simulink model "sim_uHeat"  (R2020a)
settings: Solver=ode15s  StartTime=0.0  StopTime=tsim  MaxStep=1  RelTol=1e-3
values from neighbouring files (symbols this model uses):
  dnom = [T0nom; TDnom; qDnom; Qnom]    [runTransformedMVs.m]
  Kc = 1./(tauC+theta)    [runTransformedMVs.m]
  p1 = [V1;V2;rho;cp;A1;A2;tau01; tau02;transf1]    [runTransformedMVs.m]
  p2 = [V1;V2;rho;cp;A1;A2;tau01; tau02;transf2]    [runTransformedMVs.m]
  T2nom = 30    [runTransformedMVs.m]
  tauI = 4.*(tauC+theta)    [runTransformedMVs.m]
  Tnom = [T1nom;T2nom]    [runTransformedMVs.m]
  umax = 3*Qnom    (= 5016)    [runTransformedMVs.m]
  vbias = [0;0]    [runTransformedMVs.m]
undefined symbols (not defined in the file or in its folder): CalcBlock1, CalcBlock2, Tank

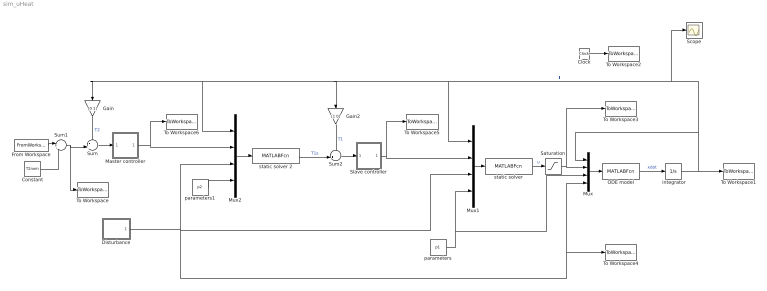
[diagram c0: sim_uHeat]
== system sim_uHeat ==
  " integrator" : Integrator  InitialCondition=Tnom
  Clock : Clock
  Constant : Constant  Value=T2nom
  Disturbance : Subsystem
  From Workspace : FromWorkspace  VariableName=T2sp  OutputAfterFinalValue=Setting to zero
  Gain : Gain  Gain=[0 1]  Multiplication=Matrix(K*u)
  Gain2 : Gain  Gain=[1 0]  Multiplication=Matrix(K*u)
  Master controller : Subsystem
  Mux : Mux
  Mux1 : Mux
  Mux2 : Mux
  ODE model : MATLABFcn  MATLABFcn=Tank(u(1:2), u(3),u(4:12),u(13:16))  OutputDimensions=2
  Saturation : Saturate  UpperLimit=umax  LowerLimit=0
  Scope : Scope
  Slave controller : Subsystem
  Sum : Sum  Inputs=-+|
  Sum1 : Sum  Inputs=|++
  Sum2 : Sum  Inputs=-+|
  To Workspace : ToWorkspace  VariableName=Tsp  SampleTime=-1
  To Workspace1 : ToWorkspace  VariableName=T  SampleTime=-1
  To Workspace2 : ToWorkspace  VariableName=time  SampleTime=-1
  To Workspace3 : ToWorkspace  VariableName=u  SampleTime=-1
  To Workspace4 : ToWorkspace  VariableName=d  SampleTime=-1
  To Workspace5 : ToWorkspace  VariableName=v1  SampleTime=-1
  To Workspace6 : ToWorkspace  VariableName=v2  SampleTime=-1
  parameters : Constant  Value=p1
  parameters1 : Constant  Value=p2
  static solver : MATLABFcn  MATLABFcn=CalcBlock1(u(1:2),u(3),u(4:7),u(8:16))  OutputDimensions=1
  static solver 2 : MATLABFcn  MATLABFcn=CalcBlock2(u(1:2),u(3),u(4:7),u(8:16))  OutputDimensions=1
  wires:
  " integrator"/1 -> Mux/1, Scope/1, Gain/1, Mux2/1, Gain2/1, Mux1/1, To Workspace1/1  "T"
  Mux/1 -> ODE model/1
  Clock/1 -> To Workspace2/1
  static solver/1 -> Saturation/1  "u"
  Mux1/1 -> static solver/1
  ODE model/1 -> " integrator"/1  "xdot"
  parameters/1 -> Mux/3, Mux1/4
  Saturation/1 -> Mux/2, To Workspace3/1
  Disturbance/1(d) -> To Workspace4/1, Mux/4, Mux1/3, Mux2/3
  Mux2/1 -> static solver 2/1
  static solver 2/1 -> Sum2/2  "T1s"
  Sum/1 -> Master controller/1(In1)
  Master controller/1(Out1) -> Mux2/2, To Workspace6/1
  Sum2/1 -> Slave controller/1(In1)
  Slave controller/1(Out1) -> Mux1/2, To Workspace5/1
  Sum1/1 -> Sum/2, To Workspace/1
  Gain/1 -> Sum/1  "T2"
  Gain2/1 -> Sum2/1  "T1"
  parameters1/1 -> Mux2/4
  From Workspace/1 -> Sum1/1
  Constant/1 -> Sum1/2

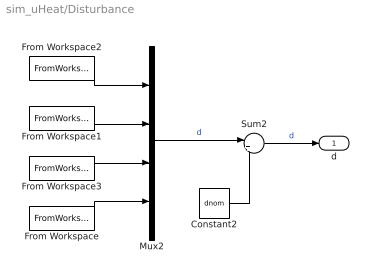
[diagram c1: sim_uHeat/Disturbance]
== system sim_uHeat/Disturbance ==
  Constant2 : Constant  Value=dnom
  From Workspace : FromWorkspace  VariableName=dist{4}  OutputAfterFinalValue=Setting to zero
  From Workspace1 : FromWorkspace  VariableName=dist{2}  OutputAfterFinalValue=Setting to zero
  From Workspace2 : FromWorkspace  VariableName=dist{1}  OutputAfterFinalValue=Setting to zero
  From Workspace3 : FromWorkspace  VariableName=dist{3}  OutputAfterFinalValue=Setting to zero
  Mux2 : Mux
  Sum2 : Sum  Inputs=|++
  d : Outport
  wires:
  From Workspace2/1 -> Mux2/1
  From Workspace/1 -> Mux2/4
  From Workspace3/1 -> Mux2/3
  Mux2/1 -> Sum2/1  "d"
  Constant2/1 -> Sum2/2
  From Workspace1/1 -> Mux2/2
  Sum2/1 -> d/1  "d"

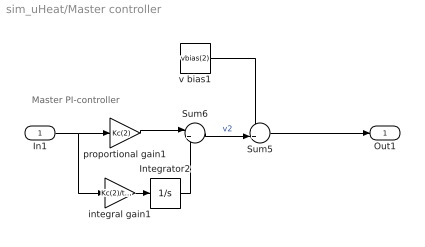
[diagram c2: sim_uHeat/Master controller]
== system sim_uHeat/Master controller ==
  note: Master PI-controller
  In1 : Inport
  Integrator2 : Integrator
  Sum5 : Sum  Inputs=++|
  Sum6 : Sum  Inputs=|++
  integral gain1 : Gain  Gain=Kc(2)/tauI(2)  Multiplication=Matrix(K*u)
  proportional gain1 : Gain  Gain=Kc(2)  Multiplication=Matrix(K*u)
  v bias1 : Constant  Value=vbias(2)
  Out1 : Outport
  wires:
  proportional gain1/1 -> Sum6/1
  Sum6/1 -> Sum5/2  "v2"
  Integrator2/1 -> Sum6/2
  In1/1 -> integral gain1/1, proportional gain1/1
  integral gain1/1 -> Integrator2/1
  Sum5/1 -> Out1/1
  v bias1/1 -> Sum5/1

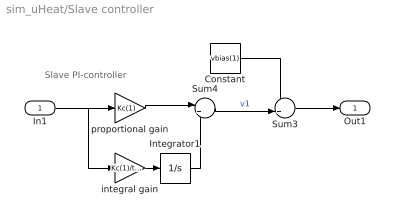
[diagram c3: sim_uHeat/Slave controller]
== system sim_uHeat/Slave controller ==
  note: Slave PI-controller
  In1 : Inport
  Constant : Constant  Value=vbias(1)
  Integrator1 : Integrator
  Sum3 : Sum  Inputs=++|
  Sum4 : Sum  Inputs=|++
  integral gain : Gain  Gain=Kc(1)/tauI(1)  Multiplication=Matrix(K*u)
  proportional gain : Gain  Gain=Kc(1)  Multiplication=Matrix(K*u)
  Out1 : Outport
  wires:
  Integrator1/1 -> Sum4/2
  proportional gain/1 -> Sum4/1
  Sum4/1 -> Sum3/2  "v1"
  In1/1 -> integral gain/1, proportional gain/1
  Sum3/1 -> Out1/1
  integral gain/1 -> Integrator1/1
  Constant/1 -> Sum3/1
